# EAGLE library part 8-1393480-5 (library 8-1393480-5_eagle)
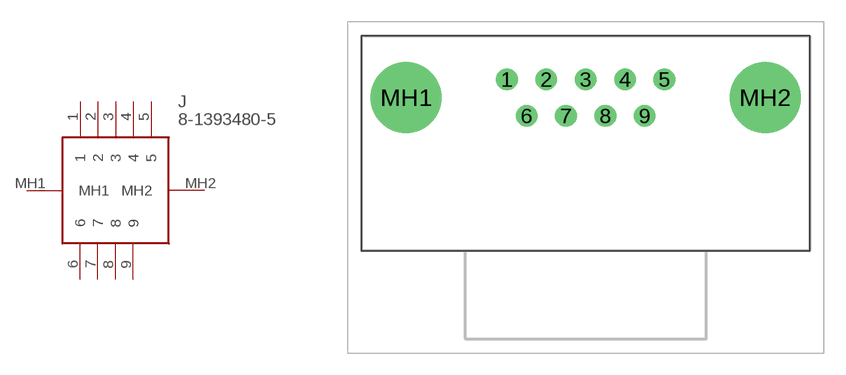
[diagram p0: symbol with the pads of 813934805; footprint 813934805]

Designator prefix J

## 8-1393480-5 (Description: 9 Way r/a Eurostyle D Plug, 4-40U Ins; Height: 12.93mm; Manufacturer_Name: TE Connectivity; Manufacturer_Part_Number: 8-1393480-5; Mouser_Part_Number: 571-8-1393480-5; Mouser_Price-Stock: https://www.mouser.co.uk/ProductDetail/TE-Connectivity-AMP/8-1393480-5?qs=tub3WQyKOl8dqJUi7eXncA%3D%3D)  [813934805]
1  1
2  2
3  3
4  4
5  5
6  6
7  7
8  8
9  9
MH1  MH1
MH2  MH2

## Footprint 813934805 (pad centres in mm)
8-1393480-5-2
drill 1 pad 1.5: 1 0,0; 2 2.74,0; 3 5.48,0; 4 8.22,0; 5 10.96,0; 6 1.37,-2.54; 7 4.11,-2.54; 8 6.85,-2.54; 9 9.59,-2.54
drill 3.3 pad 4.95: MH1 -7.02,-1.27; MH2 17.98,-1.27

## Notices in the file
This work is licensed under a Creative Commons Attribution-ShareAlike 4.0 International License (CC BY-SA) with Design Exception 1.0
